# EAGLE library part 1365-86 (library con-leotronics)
DUAL ROW STRAIGHT HEADER 1364 SERIES. 1.27mm x 1.27mm. Without Fixing Post. SMT Source: http://www.leotronics.co.uk/Conexcon/Data%20Sheets/sec.%20A/1364ing.pdf
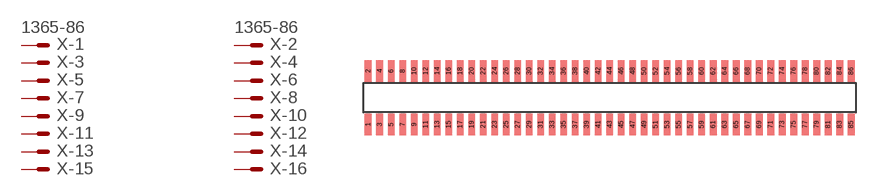
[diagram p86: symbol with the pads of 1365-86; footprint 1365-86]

Designator prefix X; gates -1=MVAL -2=MVAL -3=M -4=M -5=M -6=M -7=M -8=M -9=M -10=M -11=M -12=M -13=M -14=M -15=M -16=M -17=M -18=M -19=M -20=M -21=M -22=M -23=M -24=M -25=M -26=M -27=M -28=M -29=M -30=M -31=M -32=M -33=M -34=M -35=M -36=M -37=M -38=M -39=M -40=M -41=M -42=M -43=M -44=M -45=M -46=M -47=M -48=M -49=M -50=M -51=M -52=M -53=M -54=M -55=M -56=M -57=M -58=M -59=M -60=M -61=M -62=M -63=M -64=M -65=M -66=M -67=M -68=M -69=M -70=M -71=M -72=M -73=M -74=M -75=M -76=M -77=M -78=M -79=M -80=M -81=M -82=M -83=M -84=M -85=M -86=M

## 1365-86 (OC_FARNELL: unknown; OC_NEWARK: unknown)  [1365-86]
1  -1:S  pas
2  -2:S  pas
3  -3:S  pas
4  -4:S  pas
5  -5:S  pas
6  -6:S  pas
7  -7:S  pas
8  -8:S  pas
9  -9:S  pas
10  -10:S  pas
11  -11:S  pas
12  -12:S  pas
13  -13:S  pas
14  -14:S  pas
15  -15:S  pas
16  -16:S  pas
17  -17:S  pas
18  -18:S  pas
19  -19:S  pas
20  -20:S  pas
21  -21:S  pas
22  -22:S  pas
23  -23:S  pas
24  -24:S  pas
25  -25:S  pas
26  -26:S  pas
27  -27:S  pas
28  -28:S  pas
29  -29:S  pas
30  -30:S  pas
31  -31:S  pas
32  -32:S  pas
33  -33:S  pas
34  -34:S  pas
35  -35:S  pas
36  -36:S  pas
37  -37:S  pas
38  -38:S  pas
39  -39:S  pas
40  -40:S  pas
41  -41:S  pas
42  -42:S  pas
43  -43:S  pas
44  -44:S  pas
45  -45:S  pas
46  -46:S  pas
47  -47:S  pas
48  -48:S  pas
49  -49:S  pas
50  -50:S  pas
51  -51:S  pas
52  -52:S  pas
53  -53:S  pas
54  -54:S  pas
55  -55:S  pas
56  -56:S  pas
57  -57:S  pas
58  -58:S  pas
59  -59:S  pas
60  -60:S  pas
61  -61:S  pas
62  -62:S  pas
63  -63:S  pas
64  -64:S  pas
65  -65:S  pas
66  -66:S  pas
67  -67:S  pas
68  -68:S  pas
69  -69:S  pas
70  -70:S  pas
71  -71:S  pas
72  -72:S  pas
73  -73:S  pas
74  -74:S  pas
75  -75:S  pas
76  -76:S  pas
77  -77:S  pas
78  -78:S  pas
79  -79:S  pas
80  -80:S  pas
81  -81:S  pas
82  -82:S  pas
83  -83:S  pas
84  -84:S  pas
85  -85:S  pas
86  -86:S  pas

## Footprint 1365-86 (pad centres in mm)
DUAL ROW STRAIGHT HEADER 1364 SERIES. 1.27mm x 1.27mm. Without Fixing Post. SMT Source: http://www.leotronics.co.uk/Conexcon/Data%20Sheets/sec.%20A/1364ing.pdf
smd 0.76 x 2.4: 1 -26.67,-2.95; 2 -26.67,2.95; 3 -25.4,-2.95; 4 -25.4,2.95; 5 -24.13,-2.95; 6 -24.13,2.95; 7 -22.86,-2.95; 8 -22.86,2.95; 9 -21.59,-2.95; 10 -21.59,2.95; 11 -20.32,-2.95; 12 -20.32,2.95; 13 -19.05,-2.95; 14 -19.05,2.95; 15 -17.78,-2.95; 16 -17.78,2.95; 17 -16.51,-2.95; 18 -16.51,2.95; 19 -15.24,-2.95; 20 -15.24,2.95; 21 -13.97,-2.95; 22 -13.97,2.95; 23 -12.7,-2.95; 24 -12.7,2.95; 25 -11.43,-2.95; 26 -11.43,2.95; 27 -10.16,-2.95; 28 -10.16,2.95; 29 -8.89,-2.95; 30 -8.89,2.95; 31 -7.62,-2.95; 32 -7.62,2.95; 33 -6.35,-2.95; 34 -6.35,2.95; 35 -5.08,-2.95; 36 -5.08,2.95; 37 -3.81,-2.95; 38 -3.81,2.95; 39 -2.54,-2.95; 40 -2.54,2.95; 41 -1.27,-2.95; 42 -1.27,2.95; 43 0,-2.95; 44 0,2.95; 45 1.27,-2.95; 46 1.27,2.95; 47 2.54,-2.95; 48 2.54,2.95; 49 3.81,-2.95; 50 3.81,2.95; 51 5.08,-2.95; 52 5.08,2.95; 53 6.35,-2.95; 54 6.35,2.95; 55 7.62,-2.95; 56 7.62,2.95; 57 8.89,-2.95; 58 8.89,2.95; 59 10.16,-2.95; 60 10.16,2.95; 61 11.43,-2.95; 62 11.43,2.95; 63 12.7,-2.95; 64 12.7,2.95; 65 13.97,-2.95; 66 13.97,2.95; 67 15.24,-2.95; 68 15.24,2.95; 69 16.51,-2.95; 70 16.51,2.95; 71 17.78,-2.95; 72 17.78,2.95; 73 19.05,-2.95; 74 19.05,2.95; 75 20.32,-2.95; 76 20.32,2.95; 77 21.59,-2.95; 78 21.59,2.95; 79 22.86,-2.95; 80 22.86,2.95; 81 24.13,-2.95; 82 24.13,2.95; 83 25.4,-2.95; 84 25.4,2.95; 85 26.67,-2.95; 86 26.67,2.95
